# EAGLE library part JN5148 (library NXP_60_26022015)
IEEE802.15.4 Wireless Microcontroller The JN5148-001 is an ultra low power, high performance wireless microcontroller targeted at JenNet and ZigBee PRO networking applications. The device features an enhanced 32-bit RISC processor offering high coding efficiency through variable width instructions, a multistage instruction pipeline and low power operation with programmable clock speeds. It also includes a 2.4GHz IEEE802.15.4 compliant transceiver, 128kB of ROM, 128kB of RAM, and a rich mix of analogue and digital peripherals. The large memory footprint allows the device to run both a network stack (e.g. ZigBee PRO) and an embedded application or in a coprocessor mode. The operating current is below 18mA, allowing operation direct from a coin cell. Enhanced peripherals include low power pulse counters running in sleep mode designed for pulse counting in AMR applications and a unique Time of Flight ranging engine, allowing accurate location services to be implemented on wireless sensor networks. It also includes a 4-wire I2S audio interface, to interface directly AAL Eindhoven MK
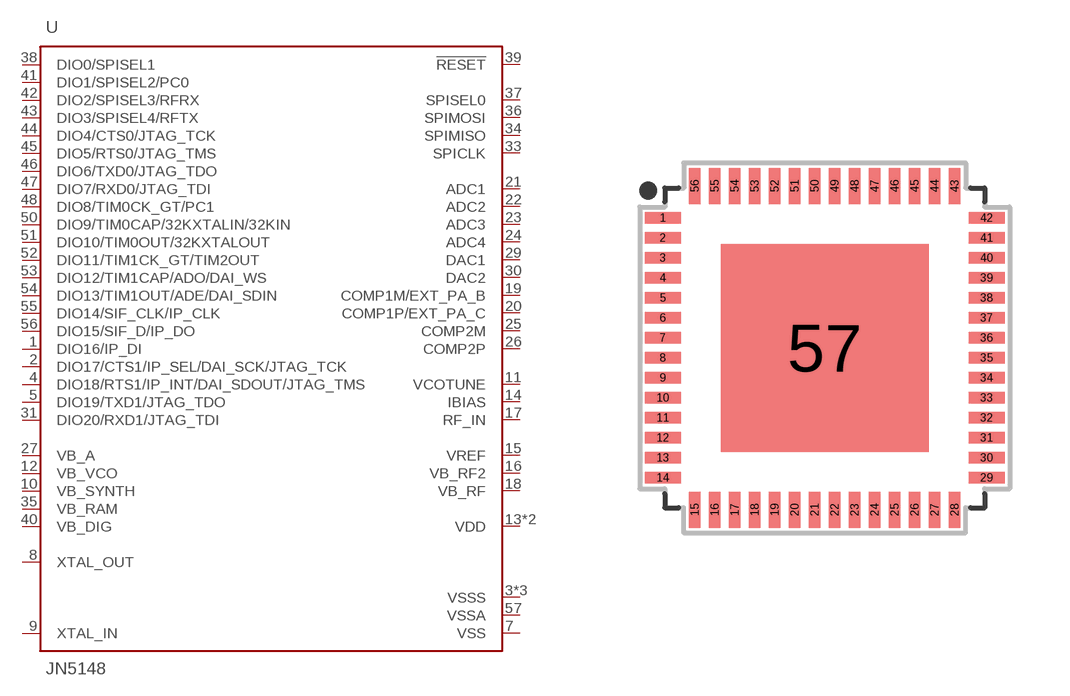
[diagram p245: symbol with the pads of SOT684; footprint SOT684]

Designator prefix U

## JN5148  [SOT684]
1  DIO16/IP_DI
2  DIO17/CTS1/IP_SEL/DAI_SCK/JTAG_TCK
3  VSSS
4  DIO18/RTS1/IP_INT/DAI_SDOUT/JTAG_TMS
5  DIO19/TXD1/JTAG_TDO
6  VSSS
7  VSS  pwr
8  XTAL_OUT  out
9  XTAL_IN  in
10  VB_SYNTH  pwr
11  VCOTUNE  pas
12  VB_VCO  pwr
13  VDD
14  IBIAS  pas
15  VREF  pas
16  VB_RF2  pwr
17  RF_IN  pas
18  VB_RF  pwr
19  COMP1M/EXT_PA_B  pas
20  COMP1P/EXT_PA_C  pas
21  ADC1  pas
22  ADC2  pas
23  ADC3  pas
24  ADC4  pas
25  COMP2M  pas
26  COMP2P  pas
27  VB_A  pwr
29  DAC1  pas
30  DAC2  pas
31  DIO20/RXD1/JTAG_TDI
32  VSSS
33  SPICLK  out
34  SPIMISO  in
35  VB_RAM  pwr
36  SPIMOSI  out
37  SPISEL0  out
38  DIO0/SPISEL1
39  !RESET!  in
40  VB_DIG  pwr
41  DIO1/SPISEL2/PC0
42  DIO2/SPISEL3/RFRX
43  DIO3/SPISEL4/RFTX
44  DIO4/CTS0/JTAG_TCK
45  DIO5/RTS0/JTAG_TMS
46  DIO6/TXD0/JTAG_TDO
47  DIO7/RXD0/JTAG_TDI
48  DIO8/TIM0CK_GT/PC1
49  VDD
50  DIO9/TIM0CAP/32KXTALIN/32KIN
51  DIO10/TIM0OUT/32KXTALOUT
52  DIO11/TIM1CK_GT/TIM2OUT
53  DIO12/TIM1CAP/ADO/DAI_WS
54  DIO13/TIM1OUT/ADE/DAI_SDIN
55  DIO14/SIF_CLK/IP_CLK
56  DIO15/SIF_D/IP_DO
57  VSSA  pwr

## Footprint SOT684 (pad centres in mm)
SOT684 HVQFN56: plastic thermal enhanced very thin quad flat package; no leads;56 terminals; body 8 x 8 x 0.85 mm JEDEC: MO-220 IEC: --
smd 0.9 x 0.29: 1 -4.05,3.25; 2 -4.05,2.75; 3 -4.05,2.25; 4 -4.05,1.75; 5 -4.05,1.25; 6 -4.05,0.75; 7 -4.05,0.25; 8 -4.05,-0.25; 9 -4.05,-0.75; 10 -4.05,-1.25; 11 -4.05,-1.75; 12 -4.05,-2.25; 13 -4.05,-2.75; 14 -4.05,-3.25; 29 4.05,-3.25; 30 4.05,-2.75; 31 4.05,-2.25; 32 4.05,-1.75; 33 4.05,-1.25; 34 4.05,-0.75; 35 4.05,-0.25; 36 4.05,0.25; 37 4.05,0.75; 38 4.05,1.25; 39 4.05,1.75; 40 4.05,2.25; 41 4.05,2.75; 42 4.05,3.25
smd 0.29 x 0.9: 15 -3.25,-4.05; 16 -2.75,-4.05; 17 -2.25,-4.05; 18 -1.75,-4.05; 19 -1.25,-4.05; 20 -0.75,-4.05; 21 -0.25,-4.05; 22 0.25,-4.05; 23 0.75,-4.05; 24 1.25,-4.05; 25 1.75,-4.05; 26 2.25,-4.05; 27 2.75,-4.05; 28 3.25,-4.05; 43 3.25,4.05; 44 2.75,4.05; 45 2.25,4.05; 46 1.75,4.05; 47 1.25,4.05; 48 0.75,4.05; 49 0.25,4.05; 50 -0.25,4.05; 51 -0.75,4.05; 52 -1.25,4.05; 53 -1.75,4.05; 54 -2.25,4.05; 55 -2.75,4.05; 56 -3.25,4.05
smd 5.2 x 5.2: 57 0,0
